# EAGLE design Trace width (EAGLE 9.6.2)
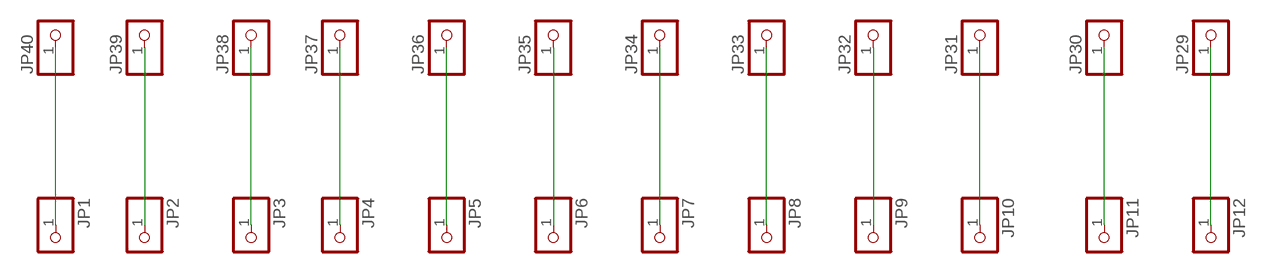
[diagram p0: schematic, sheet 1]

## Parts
JP1  PINHD-1X1  [1X01]
JP2  PINHD-1X1  [1X01]
JP3  PINHD-1X1  [1X01]
JP4  PINHD-1X1  [1X01]
JP5  PINHD-1X1  [1X01]
JP6  PINHD-1X1  [1X01]
JP7  PINHD-1X1  [1X01]
JP8  PINHD-1X1  [1X01]
JP9  PINHD-1X1  [1X01]
JP10  PINHD-1X1  [1X01]
JP11  PINHD-1X1  [1X01]
JP12  PINHD-1X1  [1X01]
JP29  PINHD-1X1  [1X01]
JP30  PINHD-1X1  [1X01]
JP31  PINHD-1X1  [1X01]
JP32  PINHD-1X1  [1X01]
JP33  PINHD-1X1  [1X01]
JP34  PINHD-1X1  [1X01]
JP35  PINHD-1X1  [1X01]
JP36  PINHD-1X1  [1X01]
JP37  PINHD-1X1  [1X01]
JP38  PINHD-1X1  [1X01]
JP39  PINHD-1X1  [1X01]
JP40  PINHD-1X1  [1X01]

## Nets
N$1: JP1.1 JP40.1
N$2: JP2.1 JP39.1
N$3: JP3.1 JP38.1
N$4: JP4.1 JP37.1
N$5: JP5.1 JP36.1
N$6: JP6.1 JP35.1
N$7: JP7.1 JP34.1
N$8: JP8.1 JP33.1
N$9: JP9.1 JP32.1
N$10: JP10.1 JP31.1
N$11: JP11.1 JP30.1
N$12: JP12.1 JP29.1

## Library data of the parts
JP1-JP12 JP29-JP40 = pinhead:PINHD-1X1: PIN HEADER

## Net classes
0 default: clearance 0.205 mm

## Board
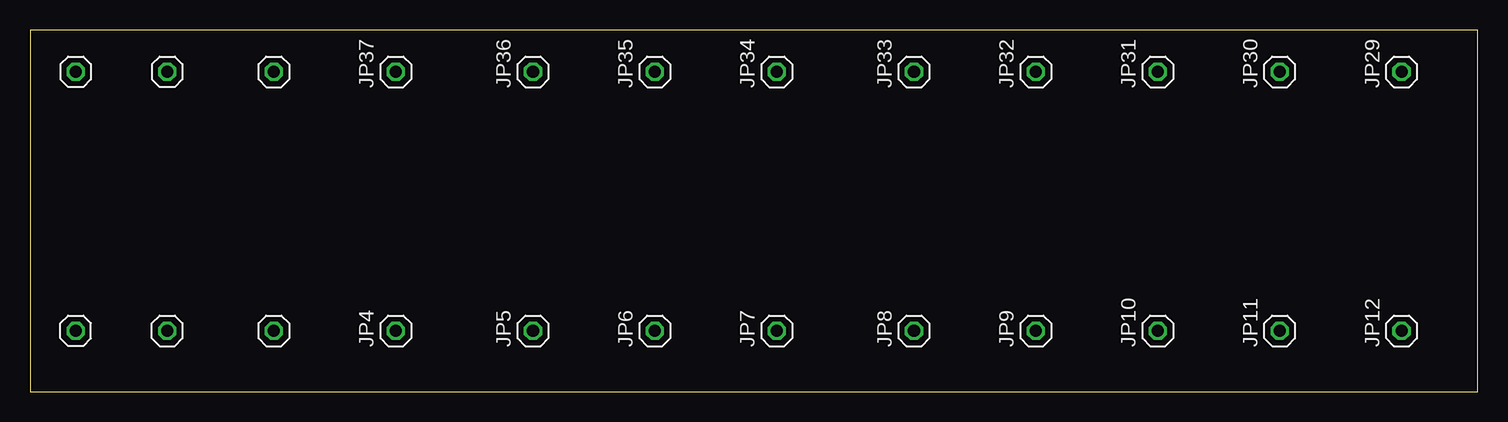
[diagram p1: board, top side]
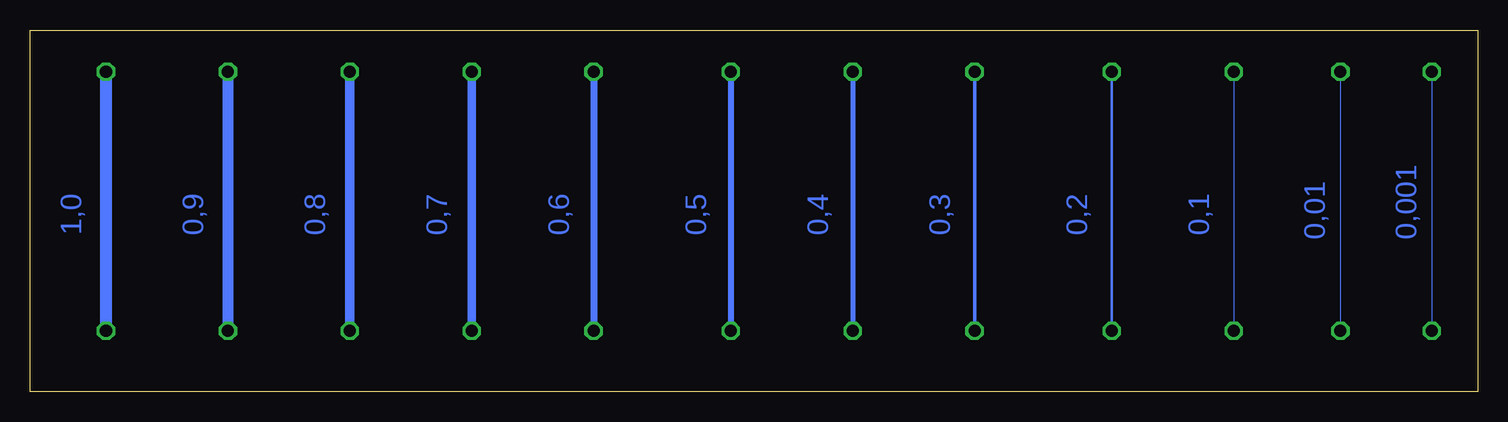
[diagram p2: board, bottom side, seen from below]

Size 120.63 x 30.15 mm. Coordinates in mm from the lower left corner, seen from the top.
Outline: 0,0 120.63,0 120.63,30.15 0,30.15 0,0
Copper layers (1*16): Top 0.035mm / dielectric 1.5mm / Bottom 0.035mm
Design rules "default": minimum track width 6mil, minimum drill 0.35mm, track to track 6mil, track to pad 6mil, pad to pad 6mil, via to via 6mil, smd to smd 6mil, copper to edge 40mil, drill to drill 6mil, minimum pad ring 10mil, minimum via ring 8mil, stop-mask expansion 4mil, vias tented up to drill 0mil, thermal gap 10mil

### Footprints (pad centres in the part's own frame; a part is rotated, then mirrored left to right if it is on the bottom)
1X01 = drill 1.016 octagon: 1 0,0

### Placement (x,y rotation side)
JP1  3.81,5.08 180 top
JP2  11.43,5.08 90 top
JP3  20.32,5.08 90 top
JP4  30.48,5.08 90 top
JP5  41.91,5.08 90 top
JP6  52.07,5.08 90 top
JP7  62.23,5.08 90 top
JP8  73.66,5.08 90 top
JP9  83.82,5.08 90 top
JP10  93.98,5.08 90 top
JP11  104.14,5.08 90 top
JP12  114.3,5.08 90 top
JP29  114.3,26.67 90 top
JP30  104.14,26.67 90 top
JP31  93.98,26.67 90 top
JP32  83.82,26.67 90 top
JP33  73.66,26.67 90 top
JP34  62.23,26.67 90 top
JP35  52.07,26.67 90 top
JP36  41.91,26.67 90 top
JP37  30.48,26.67 90 top
JP38  20.32,26.67 90 top
JP39  11.43,26.67 0 top
JP40  3.81,26.67 0 top

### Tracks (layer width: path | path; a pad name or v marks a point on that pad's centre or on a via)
N$1
  Bottom 0.001: JP40.1 JP1.1
N$2
  Bottom 0.01: JP39.1 JP2.1
N$3
  Bottom 0.1: JP38.1 JP3.1
N$4
  Bottom 0.2: JP37.1 JP4.1
N$5
  Bottom 0.3: JP36.1 JP5.1
N$6
  Bottom 0.4: JP35.1 JP6.1
N$7
  Bottom 0.5: JP34.1 JP7.1
N$8
  Bottom 0.6: JP33.1 JP8.1
N$9
  Bottom 0.7: JP32.1 JP9.1
N$10
  Bottom 0.8: JP31.1 JP10.1
N$11
  Bottom 0.9: JP30.1 JP11.1
N$12
  Bottom 1: JP29.1 JP12.1

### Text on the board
Bottom: 0,1 | 0,2 | 0,3 | 0,4 | 0,5 | 0,6 | 0,7 | 0,8 | 0,9 | 1,0 | 0,001 | 0,01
